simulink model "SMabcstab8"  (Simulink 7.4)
settings: Solver=ode45  StartTime=0.0  StopTime=10  MaxStep=2e-4  RelTol=1e-3
InitFcn:
  | smparamstab8
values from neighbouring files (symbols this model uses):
  Bm = 0.10    (= 0.1)    [IMabc2.m]    (also in imabcparam.m = 0.01; IMabcrun0.m = 0.01; IMabcrun1.m = 0.001; IMcur0.m = 1e-06)
  D = str2num(get(h,'string'))    [acttrcalc1.m]
  gam = 2*pi/3    (= 2.09439510239)    [IMabc2.m]    (also in IMabcf0.m; IMabcf1.m; imabcparam.m; IMabcrun0.m)
  H = 0.60    (= 0.6)    [IMabc2.m]    (also in IMcur0.m = 0.3; imdef0vec.m = 0.3; imdef1vec.m = 0.3; imdef2vec.m = 0.3)
  Lrr = [Lr   -Lm/2 -Lm/2    [IMabc2.m]    (also in IMabcf0.m = [Lr   -Lm1/2 -Lm1/2; IMabcf1.m = [Lr   -Lm1/2 -Lm1/2)
  R = str2num(get(h,'string'))    [acttrcalc1.m]    (also in IMabc2.m = diag([Rs Rs Rs Rr Rr Rr]); IMabcf0.m = diag([Rs Rs Rs Rr Rr Rr]); IMabcf1.m = diag([Rs Rs Rs Rr Rr Rr]); IMcurf0.m = diag([Rs Rs Rr Rr]))
  tc = abs(fco)    [im3phase.m]
  Vm = Vll*sqrt(2/3)    [imabcparam.m]
  wo = 2*pi*freq0    [calc0.m]    (also in IMabc2.m = 376.991118431; imabcparam.m = 376.991118431; IMabcrun0.m = 376.991118431; IMabcrun1.m = 376.991118431)
undefined symbols (not defined in the file or in its folder): ifo, L2, Labo, Laf, Lakd, Lakq, Lao, Row, TL, to, vector, vf

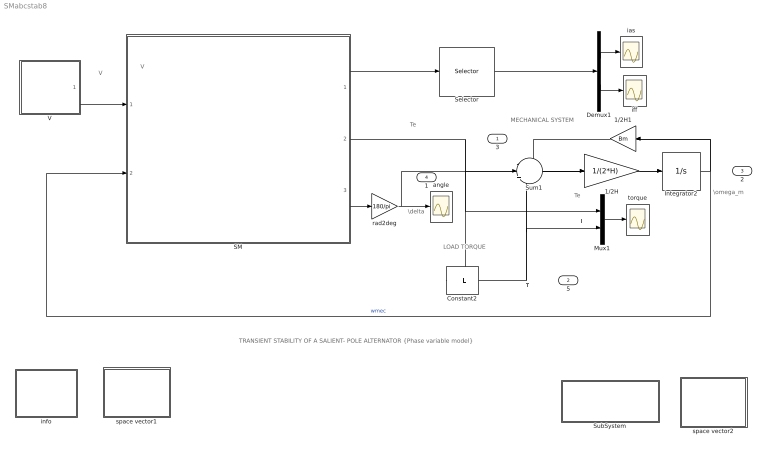
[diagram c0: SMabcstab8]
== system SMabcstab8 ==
  note: MECHANICAL SYSTEM
  note: Te
  note: Te
  note: TL
  note: LOAD TORQUE
  note: \omega_m
  note: V
  note: I
  note: \delta
  note: TL
  note: V
  note: TRANSIENT STABILITY OF A SALIENT- POLE ALTERNATOR {Phase variable model}
  1/2H : Gain  Gain=1/(2*H)  ParameterDataType=sfix(16)  ParameterScaling=2^0  OutDataType=sfix(16)  OutScaling=2^0
  1/2H1 : Gain  Gain=Bm  ParameterDataType=sfix(16)  ParameterScaling=2^0  OutDataType=sfix(16)  OutScaling=2^0
  Constant2 : Constant  Value=TL  VectorParams1D=off  OutDataType=sfix(16)  OutScaling=2^0
  Demux1 : Demux  Outputs=2
  Integrator2 : Integrator  InitialCondition=1
  Mux1 : Mux  Inputs=2
  SM : Subsystem
  Selector : Selector  InputPortWidth=6  IndexOptions=Index vector (dialog)  Indices=[1 4 ]  OutputSizes=1
  SubSystem : Subsystem
  Sum1 : Sum  Inputs=-|+|-  OutDataType=sfix(16)  OutScaling=2^0
  V : Subsystem
  angle : Scope
  ias : Scope
  iff : Scope
  info : Subsystem
  rad2deg : Gain  Gain=180/pi  ParameterDataType=sfix(16)  ParameterScaling=2^0  OutDataType=sfix(16)  OutScaling=2^0
  space vector1 : Subsystem
  space vector2 : Subsystem
  torque : Scope
  3 : Outport
  5 : Outport  Port=2
  2 : Outport  Port=3
  1 : Outport  Port=4
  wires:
  1/2H/1 -> Integrator2/1
  Integrator2/1 -> 1/2H1/1, SM/2(wm), 2/1  "wmec"
  V/1(V) -> SM/1(V)
  Sum1/1 -> 1/2H/1
  Mux1/1 -> torque/1
  Constant2/1 -> 5/1, Sum1/3, Mux1/2
  Demux1/2 -> iff/1
  Demux1/1 -> ias/1
  1/2H1/1 -> Sum1/1
  SM/1(I) -> Selector/1
  Selector/1 -> Demux1/1
  SM/2(Te) -> 3/1, Sum1/2, Mux1/1
  rad2deg/1 -> angle/1, 1/1
  SM/3(delta) -> rad2deg/1

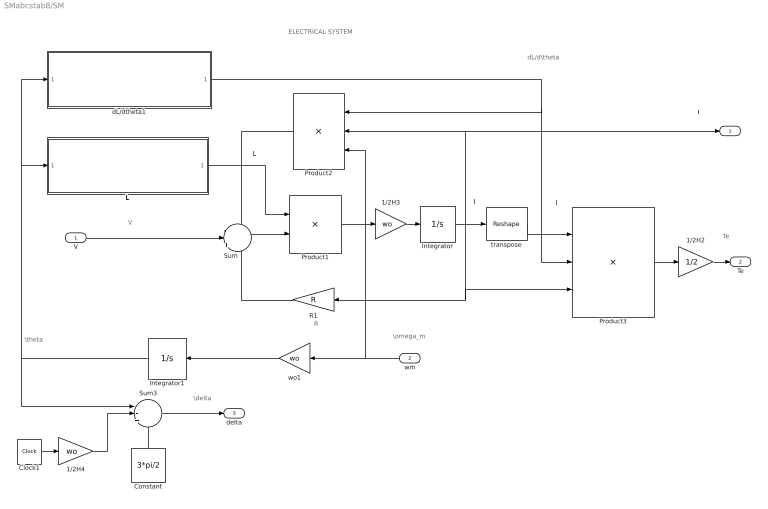
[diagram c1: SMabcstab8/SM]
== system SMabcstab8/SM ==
  note: \theta
  note: dL/d\theta
  note: L
  note: V
  note: ELECTRICAL SYSTEM
  note: I'
  note: I
  note: Te
  note: I
  note: \omega_m
  note: R
  note: \delta
  V : Inport  OutDataType=sfix(16)  OutScaling=2^0
  wm : Inport  Port=2  OutDataType=sfix(16)  OutScaling=2^0
  1/2H2 : Gain  Gain=1/2  ParameterDataType=sfix(16)  ParameterScaling=2^0  OutDataType=sfix(16)  OutScaling=2^0
  1/2H3 : Gain  Gain=wo  ParameterDataType=sfix(16)  ParameterScaling=2^0  OutDataType=sfix(16)  OutScaling=2^0
  1/2H4 : Gain  Gain=wo  ParameterDataType=sfix(16)  ParameterScaling=2^0  OutDataType=sfix(16)  OutScaling=2^0
  Clock1 : Clock
  Constant : Constant  Value=3*pi/2  OutDataType=sfix(16)  OutScaling=2^0
  Integrator : Integrator  InitialCondition="[-0.3314    0.2780    0.0534  ifo 0 0 ]'"  ZeroCross=off
  Integrator1 : Integrator  InitialCondition=5.0571
  L : Subsystem
  Product1 : Product  Inputs=/*  Multiplication=Matrix(*)  OutDataType=sfix(16)  OutScaling=2^0
  Product2 : Product  Inputs=***  Multiplication=Matrix(*)  OutDataType=sfix(16)  OutScaling=2^0
  Product3 : Product  Inputs=3  Multiplication=Matrix(*)  OutDataType=sfix(16)  OutScaling=2^0
  R1 : Gain  Gain=R  Multiplication=Matrix(K*u)  ParameterDataType=sfix(16)  ParameterScaling=2^0  OutDataType=sfix(16)  OutScaling=2^0
  Sum : Sum  Inputs=-|+|-  OutDataType=sfix(16)  OutScaling=2^0
  Sum3 : Sum  Inputs=|-++  OutDataType=sfix(16)  OutScaling=2^0
  dL/dtheta1 : Subsystem
  transpose : Reshape  OutputDimensionality=Row vector (2-D)  OutputDimensions=[1,6]
  wo1 : Gain  Gain=wo  ParameterDataType=sfix(16)  ParameterScaling=2^0  OutDataType=sfix(16)  OutScaling=2^0
  I : Outport
  Te : Outport  Port=2
  delta : Outport  Port=3
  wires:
  wo1/1 -> Integrator1/1
  R1/1 -> Sum/3
  1/2H3/1 -> Integrator/1
  Integrator/1 -> transpose/1, Product2/2, I/1, R1/1, Product3/3
  L/1(L) -> Product1/1
  Integrator1/1 -> L/1(theta), dL/dtheta1/1(theta1), Sum3/1
  Product3/1 -> 1/2H2/1
  dL/dtheta1/1(dLdtheta) -> Product2/1, Product3/2
  Product2/1 -> Sum/1
  transpose/1 -> Product3/1
  Sum/1 -> Product1/2
  Product1/1 -> 1/2H3/1
  wm/1 -> Product2/3, wo1/1
  V/1 -> Sum/2
  1/2H2/1 -> Te/1
  Clock1/1 -> 1/2H4/1
  1/2H4/1 -> Sum3/2
  Constant/1 -> Sum3/3
  Sum3/1 -> delta/1

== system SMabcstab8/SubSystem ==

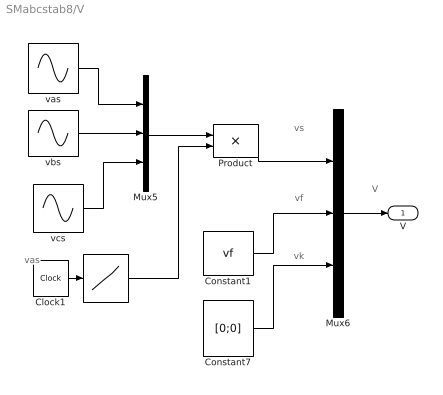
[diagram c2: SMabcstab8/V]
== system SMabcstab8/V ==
  note: vk
  note: vf
  note: vs
  note: vas
  note: V
  " " : Lookup  InputValues=[0 to to to+tc to+tc 10]  Table="[1 1 0 0  1 1]"  OutDataType=sfix(16)  OutScaling=2^0
  Clock1 : Clock
  Constant1 : Constant  Value=vf  VectorParams1D=off  OutDataType=sfix(16)  OutScaling=2^0
  Constant7 : Constant  Value=[0;0]  VectorParams1D=off  OutDataType=sfix(16)  OutScaling=2^0
  Mux5 : Mux  Inputs=3
  Mux6 : Mux  Inputs=3
  Product : Product  OutDataType=sfix(16)  OutScaling=2^0
  vas : Sin  Amplitude=Vm  Bias=0  Frequency=wo  Phase=pi/2  Samples=10  SampleTime=0
  vbs : Sin  Amplitude=Vm  Bias=0  Frequency=wo  Phase=pi/2-gam  Samples=10  SampleTime=0
  vcs : Sin  Amplitude=Vm  Bias=0  Frequency=wo  Phase=pi/2+gam  Samples=10  SampleTime=0
  V : Outport
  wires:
  Constant7/1 -> Mux6/3
  Constant1/1 -> Mux6/2
  Product/1 -> Mux6/1
  " "/1 -> Product/2
  Clock1/1 -> " "/1
  Mux5/1 -> Product/1
  vcs/1 -> Mux5/3
  vas/1 -> Mux5/1
  vbs/1 -> Mux5/2
  Mux6/1 -> V/1

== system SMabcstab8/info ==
  note: A salient pole synchronous generator is running in steady state under load when a three-phase short occurs at the terminals . A few cycles later, the fault is cleared. The dynamic equations are expressed in matrix form in terms the phase variables, namely the stator currents ias, ibs, ics; the rotor field current iff; the d-axis and q-axis damper currents idk and iqk; the anglar speed wm; and the displacement angle theta between stator as-axis and rotor direct axis. Torque, speed and current responses are plotted.The torque angle is also shown. A Matlab script file for the identical system operation is given in the file >.
  note: SYNCHRONOUS MACHINE STABILITY SALIENT POLE ROTOR (Phase variable model)

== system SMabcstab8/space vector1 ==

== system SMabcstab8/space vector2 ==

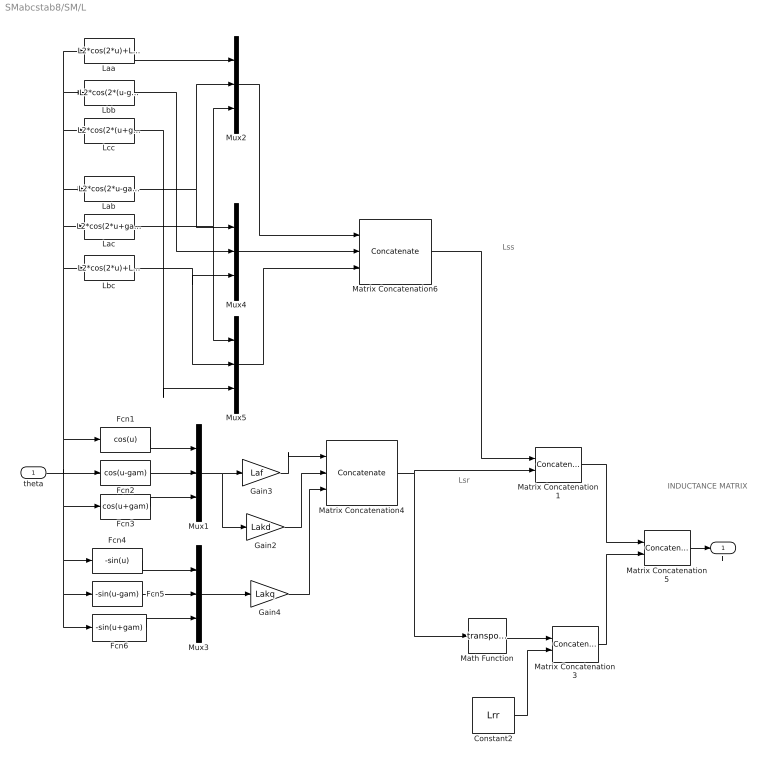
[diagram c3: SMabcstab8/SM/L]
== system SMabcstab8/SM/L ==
  note: Lsr
  note: Lss
  note: INDUCTANCE MATRIX
  theta : Inport  OutDataType=sfix(16)  OutScaling=2^0
  Constant2 : Constant  Value=Lrr  VectorParams1D=off  OutDataType=sfix(16)  OutScaling=2^0
  Fcn1 : Fcn  Expr=cos(u)
  Fcn2 : Fcn  Expr=cos(u-gam)
  Fcn3 : Fcn  Expr=cos(u+gam)
  Fcn4 : Fcn  Expr=-sin(u)
  Fcn5 : Fcn  Expr=-sin(u-gam)
  Fcn6 : Fcn  Expr=-sin(u+gam)
  Gain2 : Gain  Gain=Lakd  ParameterDataType=sfix(16)  ParameterScaling=2^0  OutDataType=sfix(16)  OutScaling=2^0
  Gain3 : Gain  Gain=Laf  ParameterDataType=sfix(16)  ParameterScaling=2^0  OutDataType=sfix(16)  OutScaling=2^0
  Gain4 : Gain  Gain=Lakq  ParameterDataType=sfix(16)  ParameterScaling=2^0  OutDataType=sfix(16)  OutScaling=2^0
  Laa : Fcn  Expr=L2*cos(2*u)+Lao
  Lab : Fcn  Expr=L2*cos(2*u-gam)+Labo
  Lac : Fcn  Expr=L2*cos(2*u+gam)+Labo
  Lbb : Fcn  Expr=L2*cos(2*(u-gam))+Lao
  Lbc : Fcn  Expr=L2*cos(2*u)+Labo
  Lcc : Fcn  Expr=L2*cos(2*(u+gam))+Lao
  Math Function : Math  Operator=transpose
  Matrix Concatenation1 : Concatenate  Mode=Multidimensional array  ConcatenateDimension=2
  Matrix Concatenation3 : Concatenate  Mode=Multidimensional array  ConcatenateDimension=2
  Matrix Concatenation4 : Concatenate  NumInputs=3  Mode=Multidimensional array  ConcatenateDimension=2
  Matrix Concatenation5 : Concatenate  Mode=Multidimensional array
  Matrix Concatenation6 : Concatenate  NumInputs=3  Mode=Multidimensional array  ConcatenateDimension=2
  Mux{1..5} (5 alike) : Mux  Inputs=3
  L : Outport
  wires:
  Matrix Concatenation6/1 -> Matrix Concatenation1/1
  Mux5/1 -> Matrix Concatenation6/3
  Mux2/1 -> Matrix Concatenation6/1
  Mux4/1 -> Matrix Concatenation6/2
  Lcc/1 -> Mux5/3
  Lbc/1 -> Mux5/2, Mux4/3
  Lac/1 -> Mux5/1, Mux2/3
  Lab/1 -> Mux4/1, Mux2/2
  Lbb/1 -> Mux4/2
  Laa/1 -> Mux2/1
  Matrix Concatenation3/1 -> Matrix Concatenation5/2
  Constant2/1 -> Matrix Concatenation3/2
  Math Function/1 -> Matrix Concatenation3/1
  Gain4/1 -> Matrix Concatenation4/3
  Mux3/1 -> Gain4/1
  Fcn6/1 -> Mux3/3
  Fcn4/1 -> Mux3/1
  Fcn5/1 -> Mux3/2
  Gain2/1 -> Matrix Concatenation4/2
  Gain3/1 -> Matrix Concatenation4/1
  theta/1 -> Lbc/1, Lac/1, Lab/1, Lcc/1, Lbb/1, Laa/1, Fcn1/1, Fcn4/1, Fcn5/1, Fcn6/1, Fcn3/1, Fcn2/1
  Fcn1/1 -> Mux1/1
  Fcn2/1 -> Mux1/2
  Fcn3/1 -> Mux1/3
  Matrix Concatenation1/1 -> Matrix Concatenation5/1
  Mux1/1 -> Gain2/1, Gain3/1
  Matrix Concatenation4/1 -> Math Function/1, Matrix Concatenation1/2
  Matrix Concatenation5/1 -> L/1

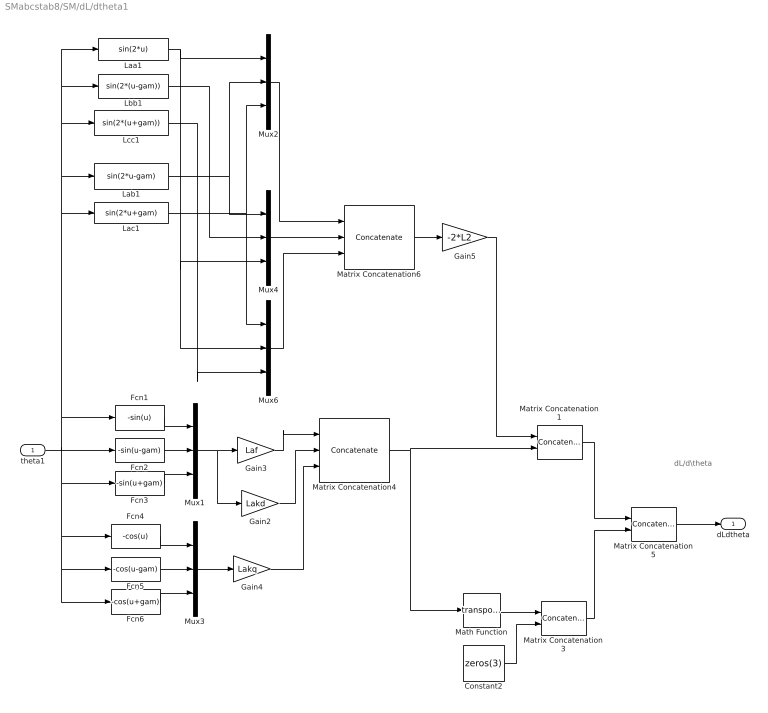
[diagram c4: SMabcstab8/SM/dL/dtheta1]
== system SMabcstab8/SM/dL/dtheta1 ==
  note: dL/d\theta
  theta1 : Inport  OutDataType=sfix(16)  OutScaling=2^0
  Constant2 : Constant  Value=zeros(3)  VectorParams1D=off  OutDataType=sfix(16)  OutScaling=2^0
  Fcn1 : Fcn  Expr=-sin(u)
  Fcn2 : Fcn  Expr=-sin(u-gam)
  Fcn3 : Fcn  Expr=-sin(u+gam)
  Fcn4 : Fcn  Expr=-cos(u)
  Fcn5 : Fcn  Expr=-cos(u-gam)
  Fcn6 : Fcn  Expr=-cos(u+gam)
  Gain2 : Gain  Gain=Lakd  ParameterDataType=sfix(16)  ParameterScaling=2^0  OutDataType=sfix(16)  OutScaling=2^0
  Gain3 : Gain  Gain=Laf  ParameterDataType=sfix(16)  ParameterScaling=2^0  OutDataType=sfix(16)  OutScaling=2^0
  Gain4 : Gain  Gain=Lakq  ParameterDataType=sfix(16)  ParameterScaling=2^0  OutDataType=sfix(16)  OutScaling=2^0
  Gain5 : Gain  Gain=-2*L2  ParameterDataType=sfix(16)  ParameterScaling=2^0  OutDataType=sfix(16)  OutScaling=2^0
  Laa1 : Fcn  Expr=sin(2*u)
  Lab1 : Fcn  Expr=sin(2*u-gam)
  Lac1 : Fcn  Expr=sin(2*u+gam)
  Lbb1 : Fcn  Expr=sin(2*(u-gam))
  Lcc1 : Fcn  Expr=sin(2*(u+gam))
  Math Function : Math  Operator=transpose
  Matrix Concatenation1 : Concatenate  Mode=Multidimensional array  ConcatenateDimension=2
  Matrix Concatenation3 : Concatenate  Mode=Multidimensional array  ConcatenateDimension=2
  Matrix Concatenation4 : Concatenate  NumInputs=3  Mode=Multidimensional array  ConcatenateDimension=2
  Matrix Concatenation5 : Concatenate  Mode=Multidimensional array
  Matrix Concatenation6 : Concatenate  NumInputs=3  Mode=Multidimensional array  ConcatenateDimension=2
  Mux{1..4,6} (5 alike) : Mux  Inputs=3
  dLdtheta : Outport
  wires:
  Gain5/1 -> Matrix Concatenation1/1
  Matrix Concatenation6/1 -> Gain5/1
  Mux6/1 -> Matrix Concatenation6/3
  Mux2/1 -> Matrix Concatenation6/1
  Mux4/1 -> Matrix Concatenation6/2
  Lcc1/1 -> Mux6/3
  Lac1/1 -> Mux6/1, Mux2/3
  Lab1/1 -> Mux4/1, Mux2/2
  Lbb1/1 -> Mux4/2
  Laa1/1 -> Mux6/2, Mux4/3, Mux2/1
  Matrix Concatenation3/1 -> Matrix Concatenation5/2
  Constant2/1 -> Matrix Concatenation3/2
  Math Function/1 -> Matrix Concatenation3/1
  Gain4/1 -> Matrix Concatenation4/3
  Mux3/1 -> Gain4/1
  Fcn6/1 -> Mux3/3
  Fcn4/1 -> Mux3/1
  Fcn5/1 -> Mux3/2
  Gain2/1 -> Matrix Concatenation4/2
  Gain3/1 -> Matrix Concatenation4/1
  theta1/1 -> Lac1/1, Lab1/1, Lcc1/1, Lbb1/1, Laa1/1, Fcn1/1, Fcn4/1, Fcn5/1, Fcn6/1, Fcn3/1, Fcn2/1
  Fcn1/1 -> Mux1/1
  Fcn2/1 -> Mux1/2
  Fcn3/1 -> Mux1/3
  Matrix Concatenation1/1 -> Matrix Concatenation5/1
  Mux1/1 -> Gain2/1, Gain3/1
  Matrix Concatenation4/1 -> Math Function/1, Matrix Concatenation1/2
  Matrix Concatenation5/1 -> dLdtheta/1
